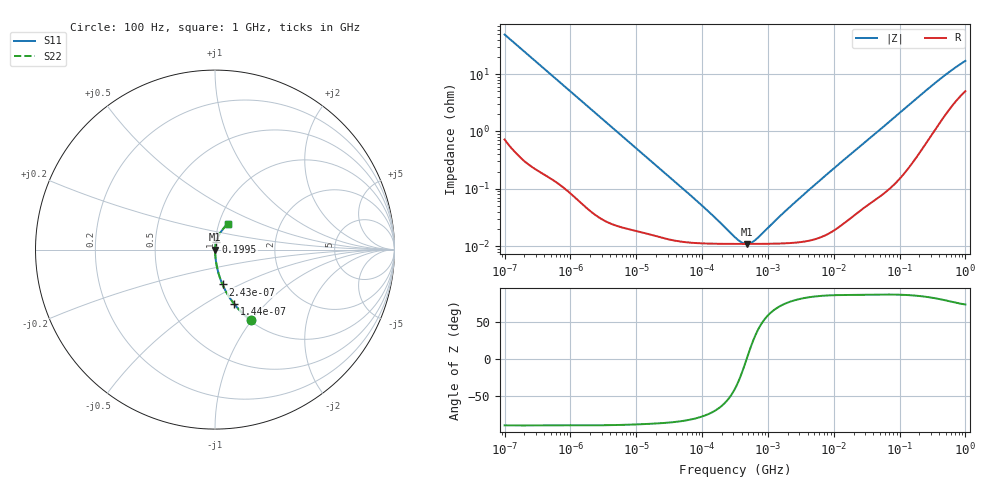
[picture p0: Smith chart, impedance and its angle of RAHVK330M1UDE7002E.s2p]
! RAHVK330M1UDE7002E  S-PARAMETER MODEL  (AEC-Q200 qualified)
! Model Generated by ELNA Corporation (http://www.ty-top.com)
! Version 1.0
! ELNA Control No. 201214
! Copyright (c) 2020 ELNA CO.,LTD. All Rights Reserved.
! Products Name : CONDUCTIVE POLYMER HYBRID ALUMINUM ELECTROLYTIC CAPACITORS
! Characteristics :
!  Capacitance  :  33uF  ,  Rated voltage  :  50V
!  Operating Temp. Range  :  -55 to +125 degC  ,  Endurance  :  4000hr at 125 degC
!  Dimension D  :  6.3mm  ,  Dimension L  :  7.7mm
! Frequency Range : 100Hz - 1GHz
! External Node Assignments :
!  1  o---| |---o  2
# MHz S RI R 50
!Freq[MHz].  S11 Real  S11 Imag  S21 Real  S21 Imag  S12 Real  S12 Imag  S22 Real  S22 Imag
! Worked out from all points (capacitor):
!   401 points, 100 Hz to 1 GHz, reference 50 ohm
!   read as one part in series: C = 32.4 uF near 108 Hz
!   lowest |Z| = 10.9 mohm at 473.2 kHz (marker M1)
!   series resonance near 476.3 kHz, so ESL is about 3.4 nH
!   S11 on the Smith chart (normalised r, x): 100 Hz: 1.01, -0.98; 144 Hz: 1.01, -0.68; 243 Hz: 1.01, -0.41; 199.5 MHz: 1.01, +0.08; 1 GHz: 1.10, +0.33
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0.0001  0.1981 -0.3913  0.8019 0.3913  0.8019 0.3913  0.1981 -0.3913
0.000144  0.1079 -0.3039  0.8921 0.3039  0.8921 0.3039  0.1079 -0.3039
0.000183  0.07 -0.2491  0.93 0.2491  0.93 0.2491  0.07 -0.2491
0.000243  0.0418 -0.1939  0.9582 0.1939  0.9582 0.1939  0.0418 -0.1939
0.000363  0.0199 -0.133  0.9801 0.133  0.9801 0.133  0.0199 -0.133
0.000543  0.00963 -0.0902  0.9904 0.0902  0.9904 0.0902  0.00963 -0.0902
0.001488  0.00168 -0.0336  0.9983 0.0336  0.9983 0.0336  0.00168 -0.0336
0.004241  0.000383 -0.0119  0.9996 0.0119  0.9996 0.0119  0.000383 -0.0119
0.022131  0.00015 -0.00231  0.9999 0.00231  0.9999 0.00231  0.00015 -0.00231
0.106537  0.000111 -0.000462  0.9999 0.000462  0.9999 0.000462  0.000111 -0.000462
0.316228  0.000109 -9.16e-05  0.9999 9.16e-05  0.9999 9.16e-05  0.000109 -9.16e-05
0.402717  0.000109 -3.67e-05  0.9999 3.67e-05  0.9999 3.67e-05  0.000109 -3.67e-05
0.473151  0.000109 -1.42e-06  0.9999 1.42e-06  0.9999 1.42e-06  0.000109 -1.42e-06
0.555904  0.000109 3.38e-05  0.9999 -3.38e-05  0.9999 -3.38e-05  0.000109 3.38e-05
0.679986  0.000109 7.92e-05  0.9999 -7.92e-05  0.9999 -7.92e-05  0.000109 7.92e-05
1.717908  0.000111 0.000362  0.9999 -0.000362  0.9999 -0.000362  0.000111 0.000362
4.704354  0.000129 0.00106  0.9999 -0.00106  0.9999 -0.00106  0.000129 0.00106
69.9842  0.00121 0.0147  0.9988 -0.0147  0.9988 -0.0147  0.00121 0.0147
199.5262  0.00581 0.0407  0.9942 -0.0407  0.9942 -0.0407  0.00581 0.0407
504.0806  0.0282 0.0917  0.9718 -0.0917  0.9718 -0.0917  0.0282 0.0917
785.2356  0.053 0.1248  0.947 -0.1248  0.947 -0.1248  0.053 0.1248
1000  0.0702 0.144  0.9298 -0.144  0.9298 -0.144  0.0702 0.144
